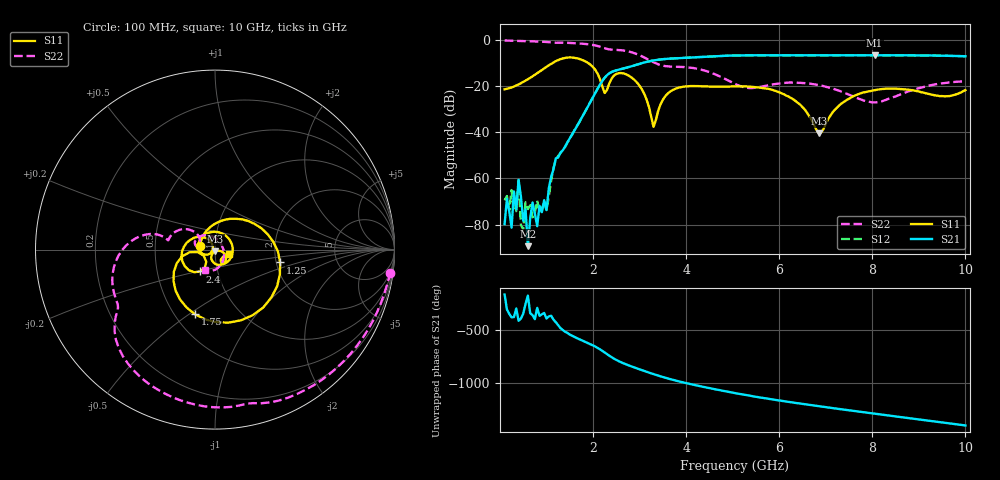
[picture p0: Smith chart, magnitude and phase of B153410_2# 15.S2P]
!  2-Port S-parameters saved by WinCal
! VAR MeasName=S-Parameters (CALIBRATED_DATA) read from VNA (N5245A)
! VAR MeasDate=2016-12-23 10:00:05
! VAR NAME=B153410_2# 15
! VAR FILENAME=B153410_2# 15.S2P
! VAR DATE=2016-12-23 10:00:05
! VAR PHYS_PORTS=1,2
# Hz S DB R 50
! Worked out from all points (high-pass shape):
!   199 points, 100 MHz to 10 GHz, reference 50 ohm
!   highest |S21| = -6.51 dB at 8.05 GHz (marker M1); lowest = -89.4 dB at 600 MHz (marker M2)
!   |S21| within 3 dB of the highest: 3.134 GHz to end of sweep
!   lowest |S11| = -40.4 dB at 6.85 GHz (marker M3), VSWR 1.02, Z = 50.2 - j0.939 ohm
!   |S11| at or under -10 dB: start of sweep to 1.124 GHz; 1.9 GHz to end of sweep
!   |S22| runs from -27.0 to -0.1 dB; largest |S21 - S12| = 0.0029
!   S11 on the Smith chart (normalised r, x): 100 MHz: 0.85, +0.04; 1.25 GHz: 2.10, -0.35; 1.75 GHz: 0.63, -0.53; 2.4 GHz: 0.82, -0.21; 10 GHz: 1.17, -0.06
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1e8  -21.35 165.3  -79.76 -164.3  -69.51 90.4  -0.13 -7.5
1.5e8  -21.07 157.6  -68.76 54.2  -67.62 140.3  -0.18 -11.0
2.5e8  -20.53 142.1  -81.34 -20.3  -65.04 -102.6  -0.25 -17.7
3e8  -20.16 134.7  -65.62 -17.5  -74.44 53.7  -0.28 -21.1
3.5e8  -19.64 127.2  -73.44 63.6  -74.15 -142.4  -0.31 -24.3
4e8  -19.23 120.4  -60.55 -52.4  -60.79 -36.1  -0.33 -27.6
4.5e8  -18.68 112.8  -67.81 -31.4  -80.15 -46.5  -0.37 -30.9
6e8  -16.96 91.4  -89.38 -174.2  -73.30 -107.8  -0.45 -40.8
1e9  -11.60 33.0  -73.73 -31.0  -73.89 -8.9  -0.79 -67.1
1.25e9  -8.64 -11.2  -50.91 -93.6  -50.27 -99.4  -1.12 -81.2
1.75e9  -8.47 -107.1  -33.88 124.4  -33.91 125.3  -1.51 -113.5
2.25e9  -22.92 -151.6  -16.29 7.6  -16.28 7.8  -3.51 -146.0
2.4e9  -16.64 -124.1  -13.81 -37.6  -13.81 -37.5  -4.12 -150.5
2.95e9  -18.52 143.1  -10.56 -144.2  -10.55 -144.3  -6.11 177.3
3.3e9  -37.62 163.0  -8.80 162.8  -8.78 162.9  -9.58 165.3
3.4e9  -30.62 -142.6  -8.49 148.7  -8.48 148.7  -10.48 165.9
5.05e9  -20.08 -4.4  -6.66 -16.6  -6.66 -16.4  -18.97 142.1
6.7e9  -34.81 -119.1  -6.57 -131.4  -6.58 -131.5  -18.99 140.1
6.85e9  -40.43 -79.8  -6.58 -140.6  -6.58 -140.7  -19.47 132.8
8.05e9  -21.71 -42.4  -6.51 148.4  -6.52 148.5  -27.01 22.5
8.35e9  -21.03 -52.4  -6.55 131.1  -6.53 131.3  -25.42 -18.1
1e10  -21.68 -18.3  -6.98 37.3  -7.00 37.6  -17.92 -117.4
